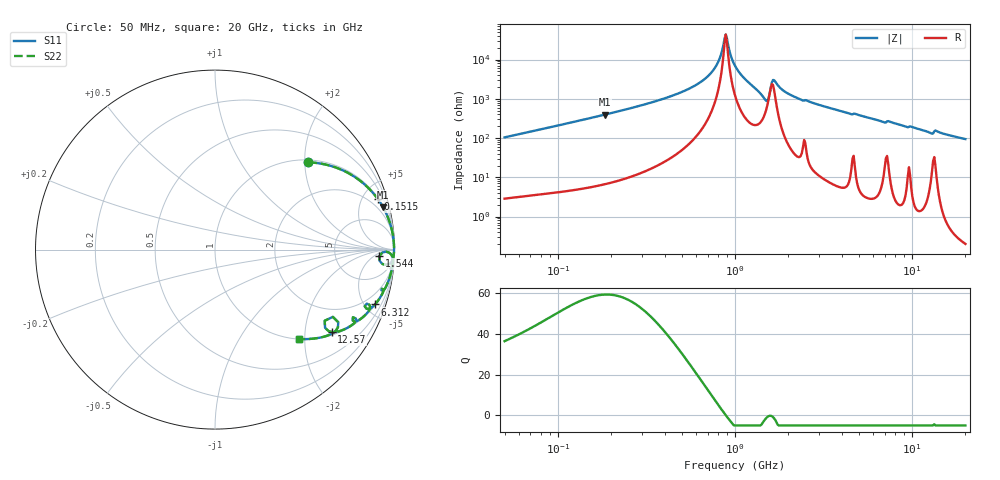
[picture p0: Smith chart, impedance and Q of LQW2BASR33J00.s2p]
!Murata Part Number: LQW2BASR33J00
!These Parameters are Measured in Series Mode Connection
!  o--[Z]--o
!Port1  Port2
!  o-------o
!Freq. Start=50[MHz] Stop=20[GHz], 401[Steps]
# Hz S RI R 50
!Freq.(Hz) S11(Real) S11(Imag) S21(Real) S21(Imag) S12(Real) S12(Imag) S22(Real) S22(Imag)
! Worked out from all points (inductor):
!   401 points, 50 MHz to 20 GHz, reference 50 ohm
!   read as one part in series: L = 330 nH near 51.52 MHz
!   highest Q = 59.2 at 184 MHz (marker M1), where L = 342 nH
!   self-resonance near 887.1 MHz
!   S11 on the Smith chart (normalised r, x): 50 MHz: 1.06, +2.08; 151.5 MHz: 1.11, +6.42; 1.544 GHz: 19, -9; 6.312 GHz: 1.06, -5.81; 12.57 GHz: 1.10, -2.75; 20 GHz: 1.00, -1.88
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5e7  0.5202 0.486  0.4798 -0.486  0.4798 -0.486  0.5202 0.486
1.364002e8  0.8879 0.3068  0.1121 -0.3068  0.1121 -0.3068  0.8879 0.3068
1.514785e8  0.9076 0.2811  0.0924 -0.2811  0.0924 -0.2811  0.9076 0.2811
1.840425e8  0.9363 0.2359  0.0637 -0.2359  0.0637 -0.2359  0.9363 0.2359
3.721004e8  0.986 0.1066  0.014 -0.1066  0.014 -0.1066  0.986 0.1066
5.411141e8  0.9946 0.0569  0.00542 -0.0569  0.00542 -0.0569  0.9946 0.0569
6.87656e8  0.997 0.0289  0.00297 -0.0289  0.00297 -0.0289  0.997 0.0289
7.868965e8  0.9976 0.0136  0.00237 -0.0136  0.00237 -0.0136  0.9976 0.0136
8.870719e8  0.9977 2.09e-05  0.00229 -2.09e-05  0.00229 -2.09e-05  0.9977 2.09e-05
1e9  0.9973 -0.0141  0.00274 0.0141  0.00274 0.0141  0.9973 -0.0141
1.110545e9  0.9962 -0.0275  0.0038 0.0275  0.0038 0.0275  0.9962 -0.0275
1.454215e9  0.9629 -0.0829  0.0371 0.0829  0.0371 0.0829  0.9629 -0.0829
1.544007e9  0.9163 -0.0357  0.0837 0.0357  0.0837 0.0357  0.9163 -0.0357
1.614971e9  0.9661 -0.015  0.0339 0.015  0.0339 0.015  0.9661 -0.015
1.664083e9  0.9811 -0.0271  0.0189 0.0271  0.0189 0.0271  0.9811 -0.0271
1.99176e9  0.991 -0.0724  0.00904 0.0724  0.00904 0.0724  0.991 -0.0724
2.728004e9  0.9821 -0.1229  0.0179 0.1229  0.0179 0.1229  0.9821 -0.1229
6.311513e9  0.8914 -0.3056  0.1086 0.3056  0.1086 0.3056  0.8914 -0.3056
7.442007e9  0.8644 -0.3202  0.1356 0.3202  0.1356 0.3202  0.8644 -0.3202
1.257102e10  0.6499 -0.459  0.3501 0.459  0.3501 0.459  0.6499 -0.459
1.396067e10  0.6746 -0.45  0.3254 0.45  0.3254 0.45  0.6746 -0.45
2e10  0.47 -0.498  0.53 0.498  0.53 0.498  0.47 -0.498
